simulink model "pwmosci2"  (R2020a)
settings: Solver=VariableStepDiscrete  StartTime=0.0  StopTime=3  FixedStep=1/44100  MaxStep=1  RelTol=1e-3  EnableMultiTasking=on
InitFcn:
  | fS = 8192;
StopFcn:
  | sound(simout.signals.values, fS);
libraries: simulink x1

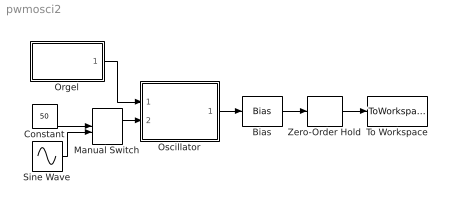
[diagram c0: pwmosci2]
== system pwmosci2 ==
  Bias : Bias  Bias=-0.5
  Constant : Constant  Value=50
  Manual Switch : ManualSwitch
  Orgel : Subsystem
  Oscillator : Subsystem  mask(PWM Oscillator){f0=400, pw0=30}
      mask prompts: f0 "Initial frequency [Hz]"; pw0 "Initial pulse width [%]"
      mask help: Oscillator producing rectangle waves of variable frequency and pulse width.
  Sine Wave : Sin  Amplitude=40  Bias=50  Frequency=2*pi*1  Phase=-pi/2  SampleTime=0
  To Workspace : ToWorkspace  VariableName=simout  SaveFormat=Structure With Time  SampleTime=-1
  Zero-Order Hold : ZeroOrderHold  SampleTime=1/fS
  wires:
  Orgel/1(Frequenz) -> Oscillator/1(In1)
  Oscillator/1(Out1) -> Bias/1
  Zero-Order Hold/1 -> To Workspace/1
  Manual Switch/1 -> Oscillator/2(In2)
  Sine Wave/1 -> Manual Switch/2
  Constant/1 -> Manual Switch/1
  Bias/1 -> Zero-Order Hold/1

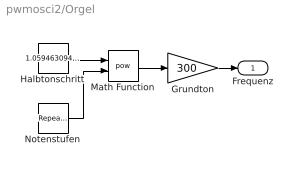
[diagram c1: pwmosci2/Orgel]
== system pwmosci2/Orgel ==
  Grundton : Gain  Gain=300
  Halbtonschritt : Constant  Value=1.059463094359295
  Math Function : Math  Operator=pow  SignedPower=on
  Notenstufen : simulink/Sources/Repeating Sequence Stair  OutValues=[12 10 12 12 12 12 12 12 12 12 12 12 10 8 7 5 4 4 4 4 5 5 5 5]  tsamp=1/8  OutMin=[]  OutMax=[]  OutDataTypeStr=double  OutputDataTypeScalingMode=double  OutDataType=fixdt(0,8)  ConRadixGroup=Best Precision: Vector-wise  OutScaling=2^-12
  Frequenz : Outport
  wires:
  Grundton/1 -> Frequenz/1
  Halbtonschritt/1 -> Math Function/1
  Notenstufen/1 -> Math Function/2
  Math Function/1 -> Grundton/1

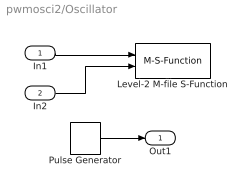
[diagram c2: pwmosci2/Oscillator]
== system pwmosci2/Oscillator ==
  In1 : Inport
  In2 : Inport  Port=2
  Level-2 M-file S-Function : M-S-Function  FunctionName=sfun_pwmosciB  Parameters=f0,pw0
  Pulse Generator : DiscretePulseGenerator  PulseType=Time based  Period=0.0016667  PulseWidth=50
  Out1 : Outport
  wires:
  In1/1 -> Level-2 M-file S-Function/1
  Pulse Generator/1 -> Out1/1
  In2/1 -> Level-2 M-file S-Function/2
